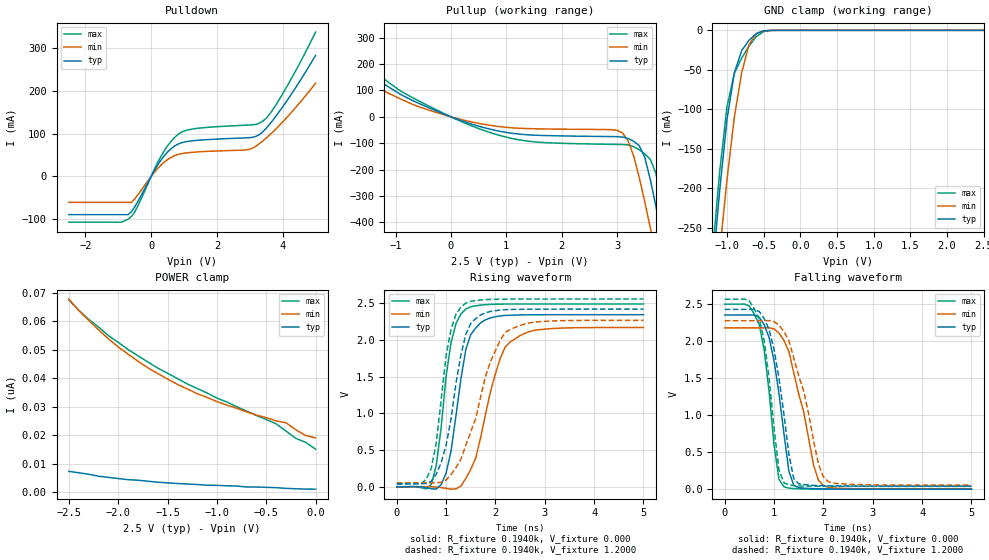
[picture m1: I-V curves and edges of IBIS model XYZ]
|   ABC Manufacturing, Inc.
|   IBIS Models for FPGA#1 device
[IBIS ver]   2.1
[File name]   abcdefg.ibs
[File Rev]   3333.3
[Date]   2/22/1905
[Source]   Hspice simulations (18-07: TT)
[Notes]   ABC IBIS model for abcdefg I/O.
   abcdefg LVDS drivers require the use of external
   resistors to provide the correct voltage levels.
   Please read ACME application note XXXXX "Abcdefg LVDS
   Drivers& Receivers:  Interface Guidelines" for details
   COMMENTS: Models include process corners for MIN and MAX.
[Disclaimer] The data in this model is derived from SPICE
simulations using modeling information extracted from the target
process. While a great deal of care has been taken to provide
information that is accurate, this model is considered preliminary
as it has not been verified by actual silicon measurement. Treat
the data in this model as preliminary until actual silicon
verification is performed.
[Copyright]   Copyright 2002, ABC Manufacturing, Inc., All rights reserved
|   Component abcdefg
[Component]   ABCDEFG
[Manufacturer]   ABC Manufacturing, Inc.
[Package]
| variable   typ   min   max
R_pkg   0.258   0.1870   0.3280
L_pkg   5.1nH   2.4000nH   7.8000nH
C_pkg   1.1pF   0.8000pF   1.4000pF
[Pin]  signal_name   model_name   R_pin   L_pin   C_pin
1   XYZ+   XYZ
2   PGND   GND
3   VCCO   POWER
| Models and submodels in the file (1): XYZ (I/O)
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|   Model XYZ
[Model]   XYZ
Model_type   I/O
Polarity   Non-Inverting
Enable   Active-Low
Vinh  = 1.4V
Vinl  = 1.0V
Vmeas =   1.2000V
Cref =  10.0000pF
Rref =   1.0000M
Vref =  0.000V
C_comp   5.0000pF   4.0000pF   6.0000pF
[Temperature Range]   25.0000   100.0000   0.000
[Voltage Range]   2.5000V   2.3750V   2.6250V
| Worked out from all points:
|   slope of the pulldown table from 0 to 0.375 V, typ, clamps not added: 8.2 ohm
|   slope of the pullup table from 0 to 0.375 V, typ, clamps not added: 13.6 ohm
|   GND clamp passes 1 mA (typ) near -0.51 V on its own axis
|   rising waveform, R_fixture 0.1940k, V_fixture 0.000: 20-80 % time 308ps typ, 476ps min, 271ps max; typ from 0 V to 2.35 V
|   rising waveform, R_fixture 0.1940k, V_fixture 1.2000: 20-80 % time 374ps typ, 616ps min, 290ps max; typ from 0.041 V to 2.42 V
|   falling waveform, R_fixture 0.1940k, V_fixture 0.000: 20-80 % time 303ps typ, 429ps min, 256ps max; typ from 2.35 V to 0 V
|   falling waveform, R_fixture 0.1940k, V_fixture 1.2000: 20-80 % time 315ps typ, 474ps min, 267ps max; typ from 2.42 V to 0.041 V
[Pulldown]
| voltage   I(typ)   I(min)   I(max)
-2.5V     -88.86mA   -60.26mA   -106.4mA
-900mV    -88.86mA   -60.26mA   -106.4mA
-600mV    -82.12mA   -60.26mA   -93.33mA
-400mV    -57.77mA   -42.35mA   -68.09mA
300mV     38.21mA    26.69mA    46.99mA
600mV     64.23mA    44.18mA    81.23mA
900mV     77.98mA    52.75mA    102.2mA
2.9V      89.95mA    61.9mA     119.6mA
3.4V      104.3mA    82.96mA    129.3mA
3.6V      121.4mA    96.48mA    144.6mA
4V        162.1mA    127mA      192.5mA
5V        282mA      217.1mA    336.2mA
[Pullup]
| voltage   I(typ)   I(min)   I(max)
-2.5V     295.5mA    231.1mA    340.7mA
-900mV    83.9mA     66.74mA    96.64mA
400mV     -29.28mA   -20.55mA   -36.46mA
1.4V      -68.49mA   -44.87mA   -92.63mA
3V        -75.36mA   -51.4mA    -104.8mA
3.2V      -82.3mA    -91.8mA    -106.8mA
3.3V      -92.74mA   -149mA     -113.1mA
3.5V      -153.5mA   -322.4mA   -140.6mA
3.6V      -237.5mA   -419.7mA   -161mA
3.8V      -446.3mA   -621.6mA   -305.8mA
4V        -670.1mA   -828.4mA   -525.3mA
5V        -1.834A    -1.888A    -1.72A
[GND_clamp]
| voltage   I(typ)   I(min)   I(max)
-2.5V     -1.803A    -1.736A    -1.828A
-1.2V     -306mA     -377.1mA   -282.8mA
-1.1V     -202.6mA   -280mA     -178.8mA
-1V       -112.6mA   -188.5mA   -96.01mA
-900mV    -53.5mA    -109.7mA   -54.54mA
-800mV    -25.67mA   -53.6mA    -35.14mA
-700mV    -12.44mA   -17.88mA   -19.83mA
-600mV    -3.983mA   -4.202mA   -7.871mA
-500mV    -601.8uA   -800.4uA   -1.51mA
-400mV    -51.06uA   -119.3uA   -124.5uA
2.5V      1.193nA    51.4nA     1.659nA
[POWER_clamp]
| voltage   I(typ)   I(min)   I(max)
-2.5V     7.392nA    67.87nA    67.52nA
-2.3V     6.403nA    60.42nA    60.77nA
-2V       4.889nA    51.05nA    52.68nA
-1.8V     4.307nA    46.04nA    47.96nA
-1.6V     3.609nA    41.73nA    43.66nA
-1.4V     3.143nA    37.95nA    39.99nA
-1V       2.503nA    31.9nA     33.12nA
-400mV    1.688nA    25.15nA    24.1nA
-300mV    1.455nA    24.45nA    21.54nA
-200mV    1.3nA      22nA       19nA
-100mV    1.2nA      20nA       17.58nA
0V        1.164nA    19.15nA    15.19nA
[Ramp]
| variable   typ   min   max
dV/dt_r   1.4070/0.3280n   1.3026/0.4908n   1.4946/0.2610n
dV/dt_f   1.4472/0.3288n   1.3535/0.4905n   1.5291/0.2665n
R_load = 0.1940k
[Rising Waveform]
R_fixture = 0.1940k
V_fixture = 0.000
| time   V(typ)   V(min)   V(max)
0s        24.75uV    13.64uV    77.86uV
700ps     -26.98mV   239.6uV    32.66mV
800ps     -32.13mV   -4.577mV   289.2mV
1ns       187.7mV    -22.82mV   1.51V
1.2ns     971.1mV    -28.25mV   2.224V
1.4ns     1.872V     113.7mV    2.422V
1.7ns     2.235V     669.4mV    2.476V
2ns       2.317V     1.542V     2.487V
2.3ns     2.338V     1.974V     2.491V
5ns       2.345V     2.171V     2.491V
[Rising Waveform]
R_fixture = 0.1940k
V_fixture = 1.2000
V_fixture_min = 1.1000
V_fixture_max = 1.3000
| time   V(typ)   V(min)   V(max)
0s        41.3mV     53.11mV    37.33mV
600ps     44.23mV    54.78mV    106.4mV
800ps     172.4mV    53.3mV     595.9mV
1ns       568.2mV    92.06mV    1.79V
1.1ns     927.4mV    167.2mV    2.144V
1.4ns     2.079V     566.9mV    2.504V
1.9ns     2.389V     1.707V     2.554V
2.2ns     2.414V     2.104V     2.557V
2.8ns     2.42V      2.245V     2.558V
5ns       2.421V     2.268V     2.558V
[Falling Waveform]
R_fixture = 0.1940k
V_fixture = 0.000
| time   V(typ)   V(min)   V(max)
0s        2.345V     2.171V     2.491V
700ps     2.316V     2.171V     2.213V
800ps     2.213V     2.172V     1.878V
1ns       1.73V      2.159V     597.4mV
1.1ns     1.29V      2.104V     131mV
1.2ns     752.5mV    2.004V     32.2mV
1.4ns     51.59mV    1.566V     8.174mV
1.8ns     6.647mV    327.1mV    2.475mV
2ns       3.765mV    48.82mV    1.564mV
5ns       206.7uV    455.5uV    236.7uV
[Falling Waveform]
R_fixture = 0.1940k
V_fixture = 1.2000
V_fixture_min = 1.1000
V_fixture_max = 1.3000
| time   V(typ)   V(min)   V(max)
0s        2.421V     2.268V     2.558V
700ps     2.393V     2.268V     2.296V
800ps     2.297V     2.269V     2.002V
1ns       1.885V     2.257V     822.7mV
1.1ns     1.494V     2.208V     254.8mV
1.2ns     1.013V     2.123V     86.57mV
1.4ns     140.8mV    1.768V     48.33mV
1.9ns     48.62mV    335.6mV    39.72mV
2.1ns     45.33mV    102.3mV    38.73mV
5ns       41.48mV    53.63mV    37.52mV
